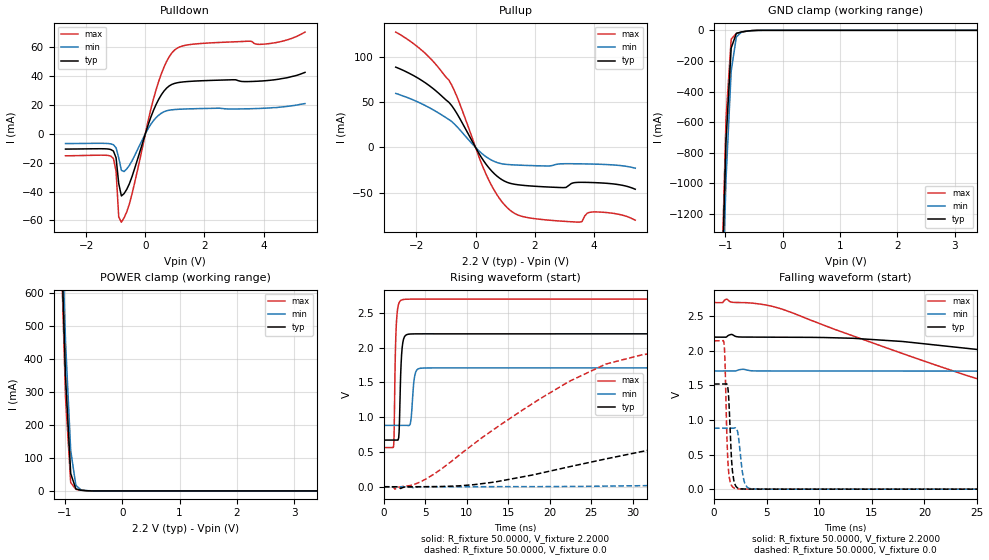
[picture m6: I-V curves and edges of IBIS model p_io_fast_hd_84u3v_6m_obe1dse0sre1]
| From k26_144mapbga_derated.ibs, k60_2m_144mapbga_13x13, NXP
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[Model] p_io_fast_hd_84u3v_6m_obe1dse0sre1
|   Model p_io_fast_hd_84u3v_6m_obe1dse0sre1
| Library cells for typ/min/max conditions are connected as defined below:
|  pad - External Pad
|  ipp_do - Core Input
|  ipp_obe - Output Buffer Enable
|  esd_boost - vdd_s_3v
|  esd_bus - vdd_s_3v
|  ipp_ina40a_3v - NC
|  ipp_ina40b_3v - NC
|  ipp_ina_3v - NC
|  ipp_ind - NC
|  ipp_ind_3v - NC
|  ipp_sre - vdd_s_lv
|  vdd_s_3v - vdd_s_3v
|  vdd_s_lv - vdd_s_lv
|  vss_bulk - vss_bulk
|  vss_s_lv - vss_s_lv
| All other pins connected to ground
Model_type I/O
Polarity   Non-Inverting
Enable   Active-High
Vinl =   0.6600V
Vinh =   1.6500V
Vmeas =  1.1000V
Cref =   25.0000pF
Rref =   50.0000
Vref =   0.0V
C_comp   3.2952pF   3.0151pF   3.6465pF
[Temperature Range]   25.0000   0.1250k   -40.0000
[Voltage Range]   2.2000V   1.7100V   2.7000V
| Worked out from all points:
|   slope of the pulldown table from 0 to 0.33 V, typ, clamps not added: 17.6 ohm
|   slope of the pullup table from 0 to 0.33 V, typ, clamps not added: 19 ohm
|   GND clamp passes 1 mA (typ) near -0.49 V on its own axis
|   POWER clamp passes 1 mA (typ) near -0.65 V on its own axis
|   rising waveform, R_fixture 50.0000, V_fixture 2.2000: 20-80 % time 244ps typ, 316ps min, 213ps max; typ from 0.671 V to 2.2 V
|   rising waveform, R_fixture 50.0000, V_fixture 0.0: 20-80 % time 43.4ns typ, 110ns min, 17.1ns max; typ from 0 V to 1.52 V
|   falling waveform, R_fixture 50.0000, V_fixture 2.2000: 20-80 % time 63ns typ, 123ns min, 28.2ns max; typ from 2.2 V to 0.673 V
|   falling waveform, R_fixture 50.0000, V_fixture 0.0: 20-80 % time 299ps typ, 408ps min, 241ps max; typ from 1.52 V to 0 V
[Pulldown]
|Voltage   I(typ)   I(min)   I(max)
-2.7V     -10.62mA   -6.81mA    -15.27mA
-1.08V    -11.96mA   -7.609mA   -17.07mA
-990mV    -16.62mA   -9.698mA   -25.88mA
-900mV    -34.47mA   -16.66mA   -57.57mA
-810mV    -43.05mA   -25.29mA   -61.23mA
-450mV    -29.63mA   -18.74mA   -41.62mA
360mV     20.13mA    11.08mA    30.28mA
720mV     31.63mA    15.91mA    50.1mA
990mV     34.87mA    16.77mA    57.99mA
1.98V     36.76mA    17.49mA    62.65mA
4.23V     37.06mA    17.9mA     62.54mA
5.4V      42.5mA     20.9mA     70.4mA
[Pullup]
|Voltage   I(typ)   I(min)   I(max)
-2.7V     88.9mA     59.8mA     127.7mA
-1.71V    71.79mA    46.54mA    104.4mA
-900mV    49.91mA    30.94mA    74.46mA
-630mV    37.51mA    23.06mA    56.23mA
360mV     -18.78mA   -10.4mA    -30.02mA
720mV     -31.59mA   -16.58mA   -52.18mA
1.17V     -39.68mA   -19.05mA   -69.56mA
2.7V      -44.11mA   -18.89mA   -81.03mA
3.51V     -38.58mA   -18.09mA   -82.69mA
3.78V     -38.65mA   -18.24mA   -72.61mA
4.05V     -38.94mA   -18.44mA   -71.34mA
5.4V      -46.22mA   -22.93mA   -80.47mA
[GND_clamp]
|Voltage   I(typ)   I(min)   I(max)
-2.7V     -32.14A    -31.92A    -32.34A
-1.08V    -1.91A     -2.124A    -1.805A
-990mV    -722.5mA   -972.4mA   -577.1mA
-900mV    -115.5mA   -266.4mA   -57.9mA
-810mV    -19.93mA   -43.77mA   -19.98mA
-720mV    -10.39mA   -11.37mA   -12.14mA
-450mV    -352.7uA   -666.6uA   -211.4uA
5.4V      0A         0A         0A
[POWER_clamp]
|Voltage   I(typ)   I(min)   I(max)
-2.7V     12.62A     12.52A     12.72A
-1.08V    845.9mA    937.2mA    801mA
-990mV    343.7mA    450.6mA    281.4mA
-900mV    52.67mA    121.9mA    25.14mA
-810mV    5.857mA    16.75mA    4.96mA
-720mV    2.026mA    3.175mA    2.02mA
-450mV    19.37uA    104.4uA    4.146uA
5.4V      0A         0A         0A
[Ramp]
| variable   typ   min   max
dV/dt_r  0.9125/43.3988n   0.5114/0.1099u   1.2875/17.0669n
dV/dt_f  0.9163/63.0526n   0.4524/0.1227u   1.2820/28.2110n
R_load = 50.0000
[Rising Waveform]
R_fixture= 50.0000
V_fixture= 2.2000
V_fixture_min= 1.7100
V_fixture_max= 2.7000
|time   V(typ)   V(min)   V(max)
0s        671.2mV    882.5mV    563.3mV
1.192ns   671.2mV    882.5mV    594.4mV
1.459ns   671.3mV    882.5mV    2.184V
1.796ns   704.1mV    882.5mV    2.629V
2.148ns   1.901V     882.5mV    2.686V
2.602ns   2.175V     882.7mV    2.697V
3.187ns   2.197V     899.2mV    2.699V
3.856ns   2.199V     1.652V     2.699V
5.053ns   2.2V       1.708V     2.699V
300ns     2.2V       1.71V      2.7V
[Rising Waveform]
R_fixture= 50.0000
V_fixture= 0.0
V_fixture_min= 0.0
V_fixture_max= 0.0
|time   V(typ)   V(min)   V(max)
0s        2.987nV    464.6nV    82.07pV
1.349ns   -5.67uV    655nV      -35.1mV
5.066ns   505.6uV    -609.5uV   109.6mV
18.88ns   194.5mV    1.806mV    1.269V
26.74ns   400.2mV    8.719mV    1.765V
42.91ns   787.4mV    51.99mV    2.043V
71.48ns   1.291V     194.7mV    2.13V
101.5ns   1.448V     357.5mV    2.143V
196.3ns   1.518V     734.2mV    2.146V
300ns     1.521V     852.4mV    2.146V
[Falling Waveform]
R_fixture= 50.0000
V_fixture= 2.2000
V_fixture_min= 1.7100
V_fixture_max= 2.7000
|time   V(typ)   V(min)   V(max)
0s        2.2V       1.71V      2.7V
6.442ns   2.199V     1.71V      2.607V
17.96ns   2.136V     1.71V      1.96V
35.59ns   1.843V     1.699V     1.135V
44.5ns    1.687V     1.684V     867.8mV
59.73ns   1.435V     1.641V     671.7mV
91.93ns   1.008V     1.52V      585.1mV
136.9ns   760.8mV    1.333V     565.5mV
221.7ns   682mV      1.067V     563.4mV
300ns     672.9mV    955.9mV    563.3mV
[Falling Waveform]
R_fixture= 50.0000
V_fixture= 0.0
V_fixture_min= 0.0
V_fixture_max= 0.0
|time   V(typ)   V(min)   V(max)
0s        1.521V     881.8mV    2.146V
940.4ps   1.521V     881.8mV    2.125V
1.027ns   1.52V      881.8mV    1.939V
1.271ns   1.504V     881.8mV    547.9mV
1.44ns    1.191V     881.8mV    182.9mV
1.868ns   136mV      882.7mV    20.98mV
2.505ns   5.861mV    507.1mV    1.276mV
2.929ns   1.863mV    82.4mV     1.131mV
3.977ns   526.6uV    1.326mV    604.5uV
300ns     91.54nV    3.546uV    1.52nV
